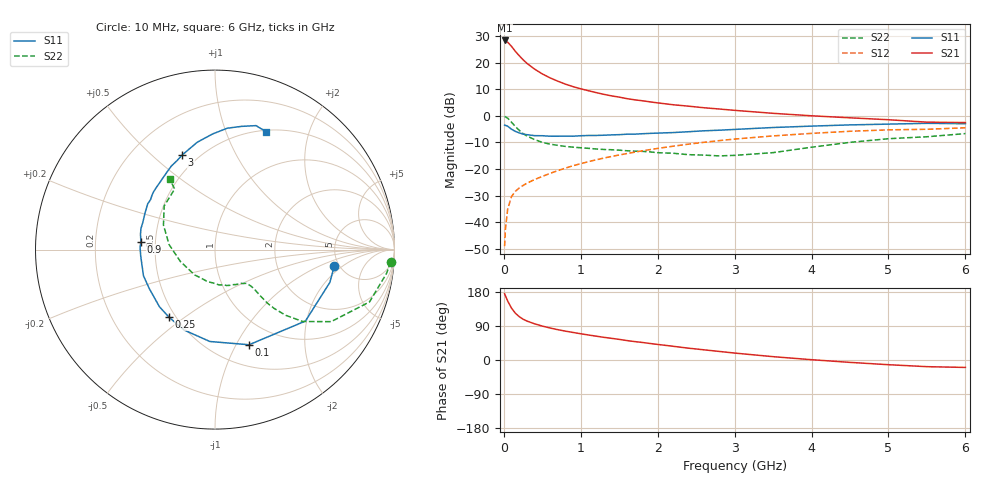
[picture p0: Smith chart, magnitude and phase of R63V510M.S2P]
! SIEMENS Small Signal Semiconductors
! BFR193
! Si NPN RF Bipolar Junction Transistor in SOT23
! VCE = 3.5 V  IC = 10 mA
! Common Emitter S-Parameters:  May  1996
# GHz  S  MA  R  50
!  f  S11  S21  S12  S22
! GHz  MAG  ANG  MAG  ANG  MAG  ANG  MAG  ANG
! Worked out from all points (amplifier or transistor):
!   36 points, 10 MHz to 6 GHz, reference 50 ohm
!   highest |S21| = 28.5 dB at 10 MHz (marker M1)
!   |S21| within 3 dB of that: start of sweep to 120.3 MHz
!   unconditionally stable (mu >= 1): 712.7 MHz to 1.997 GHz
!   at 250 MHz: K = 0.64, MSG = 23.7 dB, |S12| = -26.2 dB
!   at 1.4 GHz: K = 1.04, MAG = 10.3 dB, |S12| = -15.3 dB
!   at 6 GHz: K = 0.94, MSG = 1.0 dB, |S12| = -4.4 dB
!   lowest NFmin = 1.30 dB at 450 MHz
!   S11 on the Smith chart (normalised r, x): 10 MHz: 4.54, -1.52; 100 MHz: 0.73, -1.13; 250 MHz: 0.46, -0.44; 900 MHz: 0.41, +0.04; 3 GHz: 0.41, +0.63; 6 GHz: 0.52, +1.40
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0.01  0.6706 -7.9  26.62 174.9  0.0035 86.3  0.9816 -4.0
0.02  0.6657 -15.9  26.08 169.6  0.0072 85.5  0.9649 -7.9
0.05  0.6421 -38.3  24.64 155.6  0.0176 73.3  0.909 -18.7
0.1  0.5631 -70.3  20.59 136.8  0.0302 62.7  0.7617 -31.8
0.15  0.5128 -93.2  16.56 123.4  0.038 58.1  0.6326 -39.3
0.2  0.48 -111.0  13.74 114.4  0.0438 55.7  0.5379 -42.9
0.25  0.4557 -124.1  11.5 107.7  0.0489 55.5  0.4661 -44.8
0.3  0.4441 -134.2  9.852 102.8  0.0539 56.2  0.4192 -45.6
0.4  0.4257 -149.3  7.662 95.5  0.0633 57.6  0.3585 -45.6
0.5  0.4244 -159.9  6.219 89.5  0.0724 59.3  0.3183 -45.2
0.6  0.4157 -168.5  5.25 84.5  0.0826 61.2  0.2942 -45.3
0.7  0.4154 -175.2  4.546 80.1  0.0931 62.3  0.2793 -45.7
0.9  0.4154 173.8  3.58 72.7  0.1154 62.8  0.2581 -47.0
1.1  0.429 164.0  2.995 66.0  0.1376 63.0  0.2454 -50.5
1.3  0.4337 156.1  2.562 59.8  0.1608 62.2  0.2336 -54.3
1.6  0.4533 145.8  2.126 51.3  0.1958 60.2  0.2209 -62.1
2.2  0.4867 128.4  1.63 36.2  0.269 54.4  0.1982 -83.4
3  0.558 109.1  1.278 18.3  0.3673 43.8  0.1808 -128.3
3.5  0.6063 99.4  1.123 8.8  0.421 36.2  0.2036 -160.8
4.5  0.6795 84.3  0.924 -6.3  0.515 21.2  0.3182 154.5
5.5  0.7275 71.7  0.765 -17.6  0.5612 5.7  0.4058 123.6
6  0.7158 66.4  0.752 -19.6  0.5994 1.1  0.4657 122.8
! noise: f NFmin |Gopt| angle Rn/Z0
0.45  1.3  0.22  143  0.11
0.9  1.3  0.34  160  0.11
1.8  2.05  0.54  -153  0.14
